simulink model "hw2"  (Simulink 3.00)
settings: Solver=ode45  StartTime=0.0  StopTime=150  RelTol=1e-3
undefined symbols (not defined in the file or in its folder): K

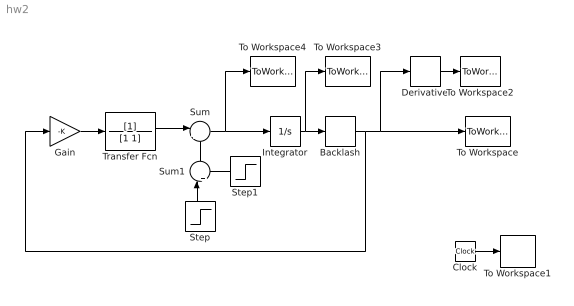
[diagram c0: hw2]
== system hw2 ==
  Backlash : Backlash  BacklashWidth=1  InitialOutput=0
  Clock : Clock
  Derivative : Derivative
  Gain : Gain  Gain=-K  SaturateOnIntegerOverflow=on
  Integrator : Integrator  ExternalReset=none  InitialConditionSource=internal  InitialCondition=0  LimitOutput=off  UpperSaturationLimit=inf  LowerSaturationLimit=-inf  ShowSaturationPort=off  ShowStatePort=off  AbsoluteTolerance=auto
  Step : Step  Orientation=up  Time=1  Before=0  After=1  SampleTime=0
  Step1 : Step  Orientation=left  Time=2  Before=0  After=1  SampleTime=0
  Sum : Sum  Inputs=|++  SaturateOnIntegerOverflow=on
  Sum1 : Sum  Orientation=up  Inputs=|+-  SaturateOnIntegerOverflow=on
  To Workspace : ToWorkspace  VariableName=th_out  SampleTime=-1  SaveFormat=Matrix
  To Workspace1 : ToWorkspace  VariableName=t  SampleTime=-1  SaveFormat=Matrix
  To Workspace2 : ToWorkspace  VariableName=dth_out  SampleTime=-1  SaveFormat=Matrix
  To Workspace3 : ToWorkspace  VariableName=th_in  SampleTime=-1  SaveFormat=Matrix
  To Workspace4 : ToWorkspace  VariableName=dth_in  SampleTime=-1  SaveFormat=Matrix
  Transfer Fcn : TransferFcn  Numerator=[1]  Denominator=[1 1]
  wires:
  Integrator/1 -> Backlash/1, To Workspace3/1
  Derivative/1 -> To Workspace2/1
  Transfer Fcn/1 -> Sum/1
  Gain/1 -> Transfer Fcn/1
  Clock/1 -> To Workspace1/1
  Backlash/1 -> Gain/1, Derivative/1, To Workspace/1
  Sum/1 -> To Workspace4/1, Integrator/1
  Step/1 -> Sum1/1
  Step1/1 -> Sum1/2
  Sum1/1 -> Sum/2
